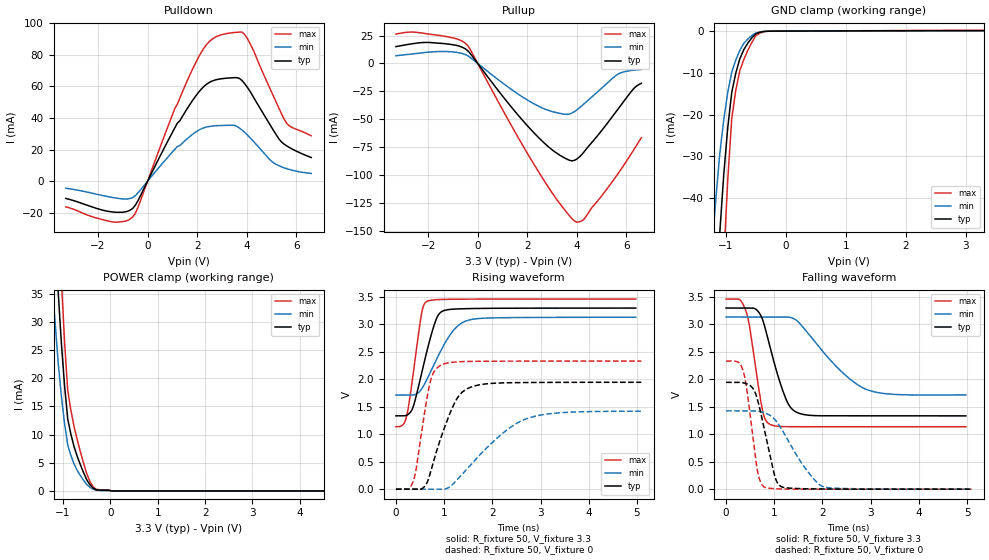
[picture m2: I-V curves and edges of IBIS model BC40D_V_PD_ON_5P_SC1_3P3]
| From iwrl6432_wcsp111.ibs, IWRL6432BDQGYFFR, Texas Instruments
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|   Model Cell BC40D_V_PD_ON_5P_SC1_3P3
|BC40D_V_PD_ON_5P_SC1_3P3
[Model]   BC40D_V_PD_ON_5P_SC1_3P3
Model_type   I/O
Polarity   Non-Inverting
Enable   Active-Low
Vinl =  0.8V
Vinh =  2V
Cref =  15pF
Rref =  100.0000M
Vref =  0V
Vmeas =  1.65
C_comp   2.059994p   1.862014p   2.067327p
|[Input load] weak_pd_on
|[Output drive] slow
|[supplytol] 5
|[temp] ind
[Model Spec]
Vinl   0.8V   0.8V   0.8V
Vinh   2V   2V   2V
[Temperature Range]   25   125   -40
[Voltage Range]   3.3   3.135   3.465
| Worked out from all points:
|   slope of the pulldown table from 0 to 0.495 V, typ, clamps not added: 31.8 ohm
|   slope of the pullup table from 0 to 0.495 V, typ, clamps not added: 33.8 ohm
|   GND clamp passes 1 mA (typ) near -0.52 V on its own axis
|   POWER clamp passes 1 mA (typ) near -0.42 V on its own axis
|   rising waveform, R_fixture 50, V_fixture 3.3: 20-80 % time 334ps typ, 511ps min, 217ps max; typ from 1.33 V to 3.3 V
|   rising waveform, R_fixture 50, V_fixture 0: 20-80 % time 466ps typ, 1.01ns min, 252ps max; typ from 0 V to 1.95 V
|   falling waveform, R_fixture 50, V_fixture 3.3: 20-80 % time 385ps typ, 889ps min, 239ps max; typ from 3.3 V to 1.33 V
|   falling waveform, R_fixture 50, V_fixture 0: 20-80 % time 293ps typ, 607ps min, 204ps max; typ from 1.95 V to 0 V
| Nom Voltages:
|   VDD=1.1, VDDS=3.3, VDDS18=1.8, ESD_BIASFET=0, VSS=0, VSSS=0
| Min Voltages:
|   VDD=1.045, VDDS=3.135, VDDS18=1.71, ESD_BIASFET=0, VSS=0, VSSS=0
| Max Voltages:
|   VDD=1.16, VDDS=3.465, VDDS18=1.89, ESD_BIASFET=0, VSS=0, VSSS=0
[POWER_clamp]
|   voltage   I(typ)   I(min)   I(max)
-3.3V     446.9mA    437.1mA    604mA
-1.233V   56.59mA    37.52mA    80.37mA
-1.167V   45.68mA    29.91mA    65.17mA
-1.1V     35.14mA    22.67mA    50.36mA
-1.033V   26.13mA    16.78mA    37.31mA
-966.7mV  18.67mA    11.95mA    26.46mA
-900mV    12.76mA    8.173mA    17.82mA
-833.3mV  10.07mA    6.293mA    14.34mA
-566.7mV  3.276mA    1.91mA     4.968mA
-366.7mV  519.9uA    314uA      774.5uA
33.33mV   0A         0A         0A
6.6V      0A         0A         0A
[Pulldown]
|   voltage   I(typ)   I(min)   I(max)
-3.3V     -10.93mA   -4.474mA   -16.27mA
-1.4V     -19.53mA   -10.38mA   -25.83mA
-600mV    -17.23mA   -10.34mA   -22.61mA
1.2V      36.72mA    21.93mA    48.76mA
1.9V      53.02mA    30.66mA    73.76mA
2.4V      61.61mA    34.34mA    86.89mA
3V        64.86mA    35.24mA    92.76mA
3.6V      65.51mA    34.65mA    94.24mA
3.9V      62.01mA    31.1mA     93.16mA
5V        34.1mA     12.57mA    56.42mA
5.6V      22.42mA    7.958mA    36.79mA
6.6V      14.97mA    4.886mA    28.74mA
[Pullup]
|   voltage   I(typ)   I(min)   I(max)
-3.3V     15.12mA    6.907mA    26.36mA
-1.9V     18.73mA    10.27mA    26.12mA
-900mV    16.4mA     10.09mA    22.38mA
-400mV    11.39mA    6.888mA    15.9mA
1.3V      -37.44mA   -22.28mA   -53.31mA
2.5V      -67.31mA   -38.74mA   -98.62mA
3.5V      -84.52mA   -45.4mA    -130.8mA
4V        -85.48mA   -41.54mA   -142.1mA
4.3V      -78.82mA   -35.86mA   -139.1mA
5.6V      -42.54mA   -10.35mA   -100.5mA
6.3V      -22.29mA   -5.95mA    -77mA
6.6V      -17.71mA   -5.359mA   -66.44mA
[GND_clamp]
|   voltage   I(typ)   I(min)   I(max)
-3.3V     -787.2mA   -627.7mA   -1.235A
-1.233V   -85.66mA   -52.14mA   -138.8mA
-1.167V   -66.47mA   -40.37mA   -107.7mA
-1.1V     -48.25mA   -29.37mA   -77.98mA
-1.033V   -34.28mA   -21.19mA   -54.56mA
-966.7mV  -23.07mA   -14.67mA   -35.51mA
-900mV    -14.62mA   -9.792mA   -20.84mA
-833.3mV  -10.07mA   -6.939mA   -14.17mA
-700mV    -4.435mA   -2.94mA    -6.836mA
-500mV    -641.2uA   -454.9uA   -1.12mA
-300mV    -31.62uA   -32.88uA   -44.11uA
3.3V      108.6uA    60.68uA    188uA
[Ramp]
| variable   typ   min   max
dV/dt_f  1.1800539/0.38506826n 0.85624661/0.8953951n  1.3975801/0.23949187n
dV/dt_r  1.1731735/0.46682557n   0.861622/1.0170237n   1.40552/0.25245197n
R_load = 50
[Rising Waveform]
R_fixture = 50
V_fixture = 3.3
V_fixture_min = 3.135
V_fixture_max = 3.465
|   time   V(typ)   V(min)   V(max)
0s        1.335V     1.713V     1.137V
145.7ps   1.335V     1.713V     1.174V
223.8ps   1.347V     1.713V     1.333V
354.7ps   1.492V     1.713V     2.079V
528.6ps   2.096V     1.819V     3.182V
642.8ps   2.515V     1.999V     3.419V
908.7ps   3.205V     2.483V     3.454V
1.202ns   3.279V     2.902V     3.459V
1.488ns   3.288V     3.073V     3.46V
4.974ns   3.298V     3.131V     3.462V
[Rising Waveform]
R_fixture = 50
V_fixture = 0
V_fixture_min = 0
V_fixture_max = 0
|   time   V(typ)   V(min)   V(max)
0s        0V         0V         0V
262.4ps   0V         0V         0V
360.3ps   0V         0V         146mV
575ps     31.96mV    0V         1.286V
707.5ps   277.4mV    0V         1.939V
931.8ps   934.1mV    0V         2.257V
1.274ns   1.661V     175.6mV    2.319V
1.626ns   1.879V     516.9mV    2.328V
2.786ns   1.943V     1.305V     2.332V
5.091ns   1.946V     1.421V     2.333V
[Falling Waveform]
R_fixture = 50
V_fixture = 3.3
V_fixture_min = 3.135
V_fixture_max = 3.465
|   time   V(typ)   V(min)   V(max)
0s        3.298V     3.134V     3.461V
276.8ps   3.298V     3.134V     3.454V
412.9ps   3.298V     3.134V     3.243V
749.7ps   3.105V     3.134V     1.462V
910.7ps   2.593V     3.134V     1.18V
1.252ns   1.623V     3.134V     1.138V
1.512ns   1.382V     3.033V     1.136V
2.315ns   1.336V     2.209V     1.136V
2.892ns   1.335V     1.823V     1.136V
4.974ns   1.334V     1.716V     1.136V
[Falling Waveform]
R_fixture = 50
V_fixture = 0
V_fixture_min = 0
V_fixture_max = 0
|   time   V(typ)   V(min)   V(max)
0s        1.945V     1.426V     2.332V
353.8ps   1.938V     1.426V     2.155V
435.7ps   1.916V     1.426V     1.789V
651.5ps   1.633V     1.422V     333.5mV
797.8ps   1.078V     1.39V      35.05mV
1.002ns   266.1mV    1.28V      8.379mV
1.101ns   74.01mV    1.165V     5.162mV
1.623ns   7.433mV    406.4mV    0V
2.007ns   3.705mV    49.22mV    0V
5.091ns   0V         0V         0V
